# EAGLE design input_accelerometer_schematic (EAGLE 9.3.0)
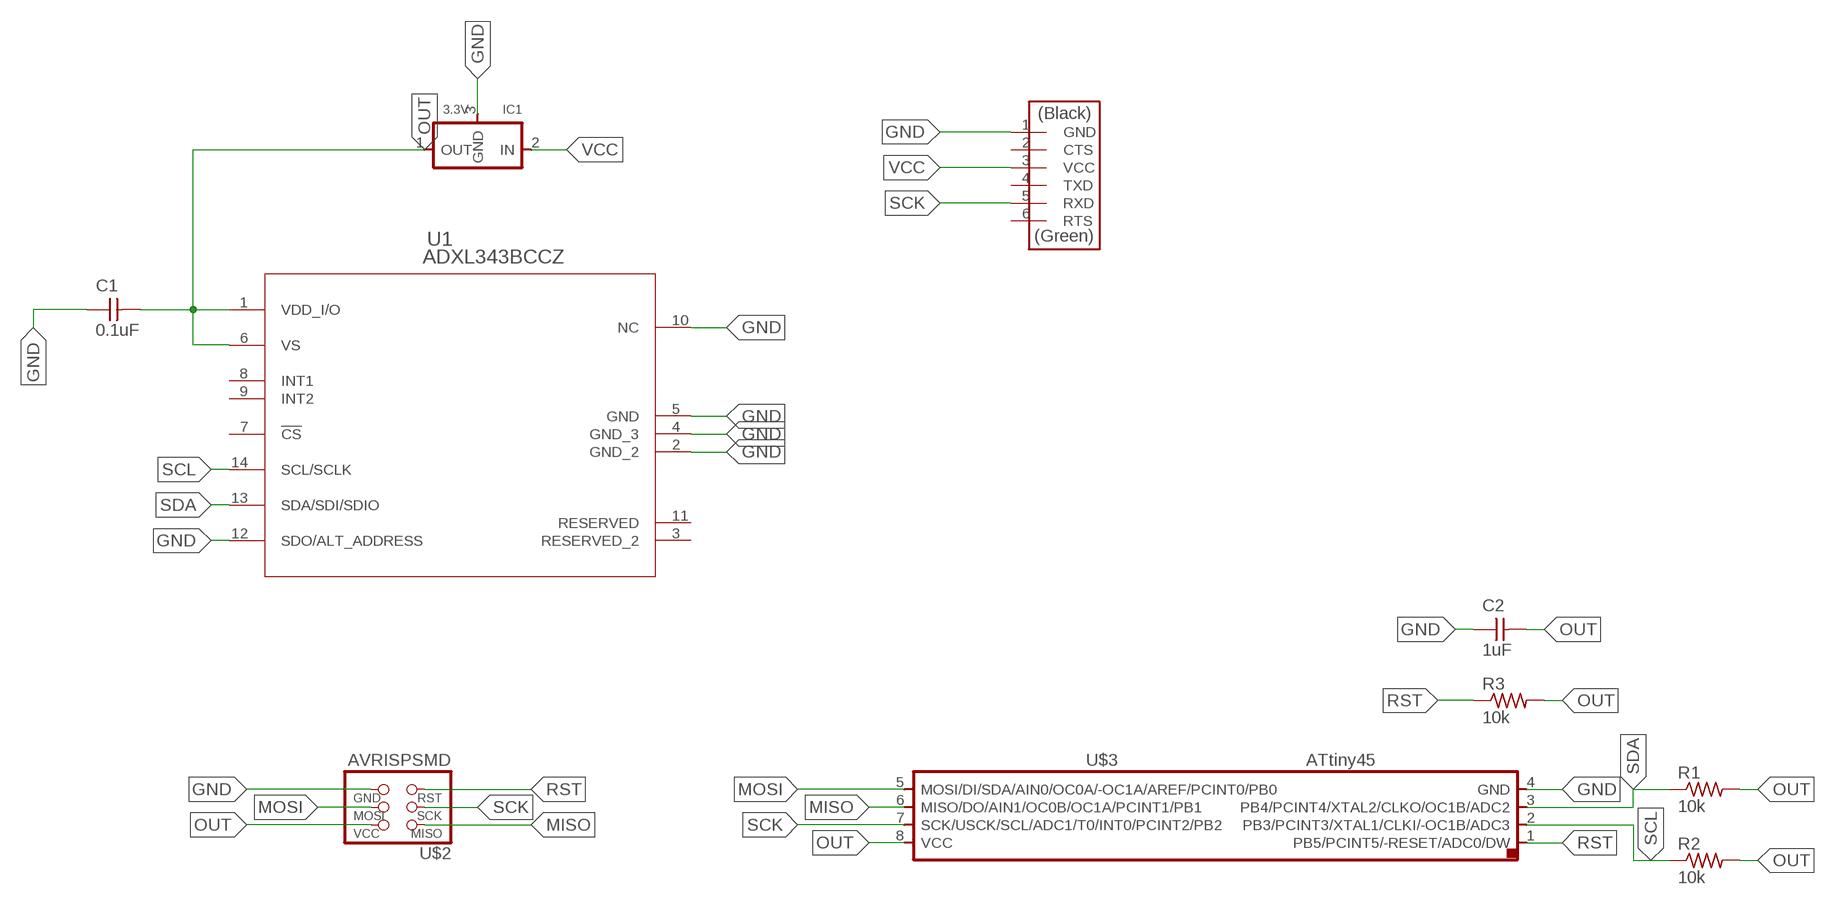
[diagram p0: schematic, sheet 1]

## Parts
C1  0.1uF  CAP-UNPOLARIZEDFAB  [C1206FAB]
C2  1uF  CAP-UNPOLARIZEDFAB  [C1206FAB]
IC1  3.3V  REGULATORSOT23  [SOT23]
R1  10k  RES-US1206FAB  [R1206FAB]
R2  10k  RES-US1206FAB  [R1206FAB]
R3  10k  RES-US1206FAB  [R1206FAB]
U1  ADXL343BCCZ  [LGA_CC-14-1]
U$1  FTDI-SMD-HEADER  [1X06SMD]
U$2  AVRISPSMD  [2X03SMD]
U$3  ATTINY45SI  [SOIC8]

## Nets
GND: C1.1 C2.1 IC1.3(GND) U1.2(GND_2) U1.4(GND_3) U1.5(GND) U1.10(NC) U1.12(SDO/ALT_ADDRESS) U$1.1(GND) U$2.6(GND) U$3.4(GND)
MISO: U$2.1(MISO) U$3.6(MISO/DO/AIN1/OC0B/OC1A/PCINT1/PB1)
MOSI: U$2.4(MOSI) U$3.5(MOSI/DI/SDA/AIN0/OC0A/-OC1A/AREF/PCINT0/PB0)
OUT: C1.2 C2.2 IC1.1(OUT) R1.2 R2.2 R3.2 U1.1(VDD_I/O) U1.6(VS) U$2.2(VCC) U$3.8(VCC)
RST: R3.1 U$2.5(RST) U$3.1(PB5/PCINT5/-RESET/ADC0/DW)
SCK: U$1.5(RXD) U$2.3(SCK) U$3.7(SCK/USCK/SCL/ADC1/T0/INT0/PCINT2/PB2)
SCL: R2.1 U1.14(SCL/SCLK) U$3.2(PB3/PCINT3/XTAL1/CLKI/-OC1B/ADC3)
SDA: R1.1 U1.13(SDA/SDI/SDIO) U$3.3(PB4/PCINT4/XTAL2/CLKO/OC1B/ADC2)
VCC: IC1.2(IN) U$1.3(VCC)
Unconnected: U1.3(RESERVED_2) U1.7(!CS) U1.8(INT1) U1.9(INT2) U1.11(RESERVED) U$1.2(CTS) U$1.4(TXD) U$1.6(RTS)

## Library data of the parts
C1 C2 = fab:CAP-UNPOLARIZED
IC1 = fab:REGULATOR
R1-R3 = fab:RES-US: Resistor (US Symbol)
U1 = adxl343:ADXL343BCCZ; MANUFACTURER_PART_NUMBER: ADXL343BCCZ; VENDOR: Analog Devices Inc
U$1 = fab:FTDI-SMD-HEADER
U$2 = fab:AVRISP
U$3 = fab:ATTINY45

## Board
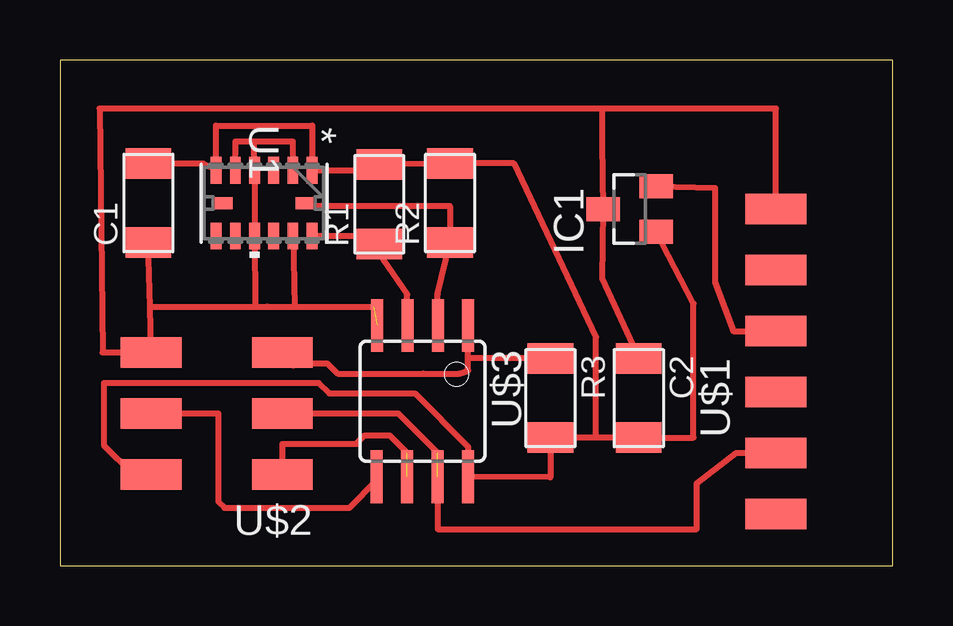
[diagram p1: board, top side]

Size 34.72 x 21.07 mm. Coordinates in mm from the lower left corner, seen from the top.
Outline: 0,0 34.72,0 34.72,21.07 0,21.07 0,0
Copper layers (1*16): Top 0.035mm / dielectric 1.5mm / Bottom 0.035mm
Design rules "fabmodule *": minimum track width 10mil, minimum drill 0.4mm, track to track 0.26mm, track to pad 0.26mm, pad to pad 0.26mm, via to via 0.26mm, smd to smd 0.26mm, copper to edge 40mil, drill to drill 0.8mm, minimum pad ring 10mil, minimum via ring 8mil, stop-mask expansion 4mil, vias tented up to drill 0mil, thermal gap 10mil

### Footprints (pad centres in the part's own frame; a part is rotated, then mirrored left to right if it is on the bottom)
C1206FAB = smd 1.27 x 1.905: 1 -1.651,0; 2 1.651,0
SOT23 = smd 1 x 1.4: 1 -0.95,-1.1; 2 0.95,-1.1; 3 0,1.1
R1206FAB = smd 1.27 x 1.905: 1 -1.651,0; 2 1.651,0
LGA_CC-14-1 = smd 1.118 x 0.449: 1 -1.371,2; 2 -1.371,1.2; 3 -1.371,0.4; 4 -1.371,-0.4; 5 -1.371,-1.2; 6 -1.371,-2; 8 1.371,-2; 9 1.371,-1.2; 10 1.371,-0.4; 11 1.371,0.4; 12 1.371,1.2; 13 1.371,2 | smd 0.5 x 0.813: 7 0,-1.718; 14 0,1.718
1X06SMD = smd 2.54 x 1.27: 1 0,6.35; 2 0,3.81; 3 0,1.27; 4 0,-1.27; 5 0,-3.81; 6 0,-6.35
2X03SMD = smd 2.54 x 1.27: 1 -2.54,2.54; 2 2.92,2.54; 3 -2.54,0; 4 2.92,0; 5 -2.54,-2.54; 6 2.92,-2.54
SOIC8 = smd 0.5 x 2.2: 1 -1.905,-3.154; 2 -0.645,-3.154; 3 0.625,-3.154; 4 1.895,-3.154; 5 1.905,3.154; 6 0.635,3.154; 7 -0.635,3.154; 8 -1.905,3.154

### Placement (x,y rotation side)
C1  3.68,15.11 90 top
C2  24.13,6.99 270 top
IC1  23.75,14.86 90 top
R1  13.31,15.06 90 top
R2  16.26,15.11 90 top
R3  20.45,6.99 270 top
U1  8.51,15.11 270 top
U$1  29.84,8.51 0 top
U$2  6.73,6.35 180 top
U$3  15.11,6.86 180 top

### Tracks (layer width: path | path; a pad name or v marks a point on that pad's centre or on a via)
GND  (1 unrouted)
  Top 0.254: C2.1 22.61,11.94 IC1.3 22.61,17.65 22.61,19.05 | U$1.1 29.84,19.05 22.61,19.05 | 22.61,19.05 1.65,19.05 1.78,8.89 U$2.6 3.76,10.8 | 3.76,10.8 C1.1 | 3.76,10.8 8.13,10.8 | 8.13,10.8 8.64,10.8 9.78,10.8 | 9.78,10.8 13.08,10.79 | 8.13,10.8 U1.10 U1.4 8.1,17.68 | U1.12 9.78,10.8 | U1.5 7.32,17.68 8.1,17.68 | 8.1,17.68 9.7,17.68 U1.2
MISO  (1 unrouted)
  Top 0.254: U$2.1 9.27,5.08 12.35,5.08 12.7,5.43 13.75,5.43 14.48,4.7
MOSI
  Top 0.254: U$2.4 6.6,6.35 6.6,2.67 6.86,2.41 12.06,2.41 13.21,3.56
  Top 0.406: 13.21,3.56 U$3.5
OUT
  Top 0.254: 3.05,3.81 1.83,5.03 1.83,7.61 10.8,7.61 11.23,7.18 14.79,7.18 17.02,4.95 U$3.8 20.45,3.68 R3.2 22.35,5.33 | IC1.1 26.42,10.92 26.42,5.33 C2.2 22.35,5.33 | 22.35,5.33 22.35,9.53 18.92,16.76 R2.2 R1.2 12.52,16.48 U1.1 10.51,16.64 10.52,18.34 6.5,18.34 U1.6 5.97,16.76 C1.2
  Top 0.406: 3.05,3.81 U$2.2
RST
  Top 0.254: 9.73,8.44 11.14,8.44 11.57,8 15.14,8 16.64,8 17.02,8.13 17.02,8.64 | 17.02,8.64 U$3.1 | R3.1 17.02,8.64
  Top 0.406: U$2.5 9.73,8.44
SCK  (1 unrouted)
  Top 0.254: U$2.3 14.1,6.35 15.75,4.7 | U$3.7 15.75,1.52 26.54,1.52 26.54,3.43 28.19,4.7 U$1.5
SCL
  Top 0.254: U1.14 10.35,14.99 16.26,14.99 R2.1 15.75,11.3 U$3.2
SDA
  Top 0.254: U$3.3 14.48,11.3 13.49,12.72 R1.1 12.65,13.74 U1.13
VCC
  Top 0.254: IC1.2 27.3,15.75 27.3,11.81 28.07,9.78 U$1.3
